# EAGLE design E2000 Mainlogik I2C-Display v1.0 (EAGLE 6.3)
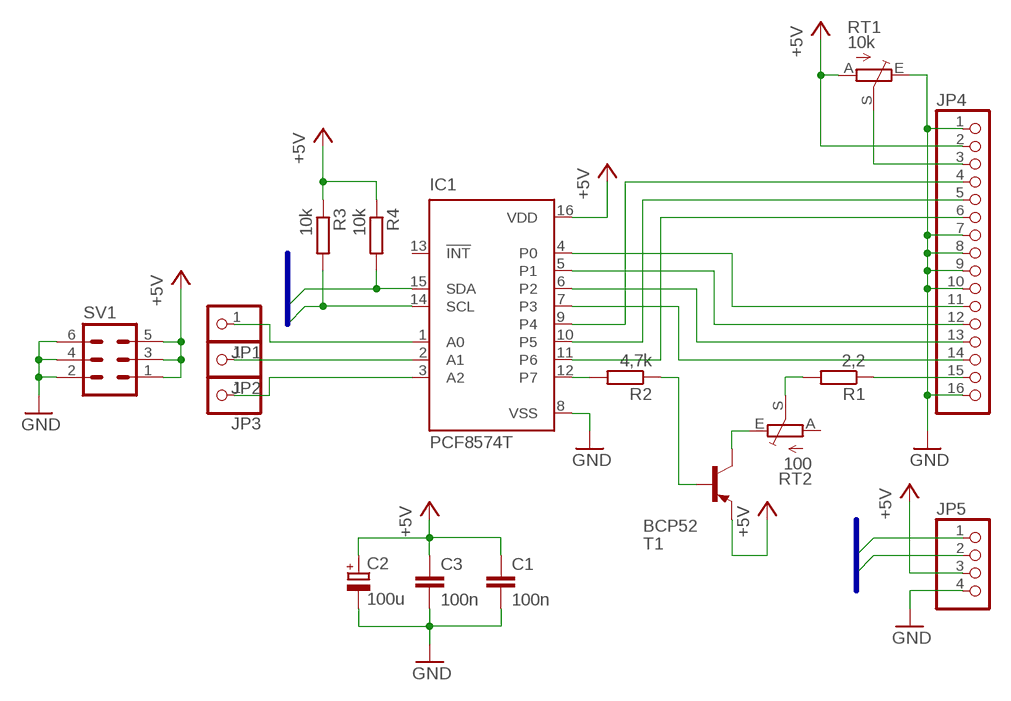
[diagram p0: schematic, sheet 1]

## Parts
C1  100n  C-EUC1206  [C1206]
C2  100u  CPOL-EUD  [PANASONIC_D]
C3  100n  C-EUC1206  [C1206]
IC1  PCF8574T  [SO16W]
JP1  PINHD-1X1  [1X01]
JP2  PINHD-1X1  [1X01]
JP3  PINHD-1X1  [1X01]
JP4  PINHD-1X16  [1X16]
JP5  PINHD-1X4  [1X04]
R1  2,2  R-EU_R1206  [R1206]
R2  4,7k  R-EU_R1206  [R1206]
R3  10k  R-EU_R1206  [R1206]
R4  10k  R-EU_R1206  [R1206]
RT1  10k  TRIM_EU-CA6V  [CA6V]
RT2  100  TRIM_EU-CA6V  [CA6V]
SV1  MA03-2  [MA03-2]
T1  BCP52  [SOT223]

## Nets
+5V: C1.1 C2.+ C3.1 IC1.16(VDD) JP4.2 JP5.3 R3.1 R4.1 RT1.A SV1.1 SV1.3 SV1.5 T1.3(E)
GND: C1.2 C2.- C3.2 IC1.8(VSS) JP4.1 JP4.7 JP4.8 JP4.9 JP4.10 JP4.16 JP5.4 RT1.E SV1.2 SV1.4 SV1.6
N$1: IC1.12(P7) R2.2
N$2: R2.1 T1.1(B)
N$3: RT2.E T1.2(C) T1.4(C)
N$4: R1.2 RT2.S
N$5: JP4.15 R1.1
N$6: IC1.9(P4) JP4.4
N$7: IC1.10(P5) JP4.5
N$8: IC1.11(P6) JP4.6
N$9: IC1.7(P3) JP4.14
N$10: IC1.6(P2) JP4.13
N$11: IC1.5(P1) JP4.12
N$12: IC1.4(P0) JP4.11
N$13: IC1.2(A1) JP2.1
N$14: JP4.3 RT1.S
N$15: IC1.3(A2) JP3.1
N$16: IC1.1(A0) JP1.1
SCL: IC1.14(SCL) JP5.1 R3.2
SDA: IC1.15(SDA) JP5.2 R4.2
Unconnected: IC1.13(!INT) RT2.A

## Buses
SDA,SCL

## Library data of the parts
C1 C3 = rcl:C-EU: CAPACITOR, European symbol
C2 = rcl:CPOL-EU: POLARIZED CAPACITOR, European symbol
IC1 = micro-philips:PCF8574: I2C-Bus Remote 8-bit I/O expander http://www.semiconductors.philips.com/acrobat_download/datasheets/PCF8574_4.pdf; MPN: PCF8574T/3,512; OC_FARNELL: 1201255; OC_NEWARK: 70R6870
JP1-JP3 = pinhead:PINHD-1X1: PIN HEADER
JP4 = pinhead:PINHD-1X16: PIN HEADER
JP5 = pinhead:PINHD-1X4: PIN HEADER
R1-R4 = rcl:R-EU_: RESISTOR, European symbol
RT1 RT2 = pot:TRIM_EU-: POTENTIOMETER
SV1 = con-lstb:MA03-2: PIN HEADER; OC_FARNELL: unknown; OC_NEWARK: unknown
T1 = transistor-pnp:BCP52

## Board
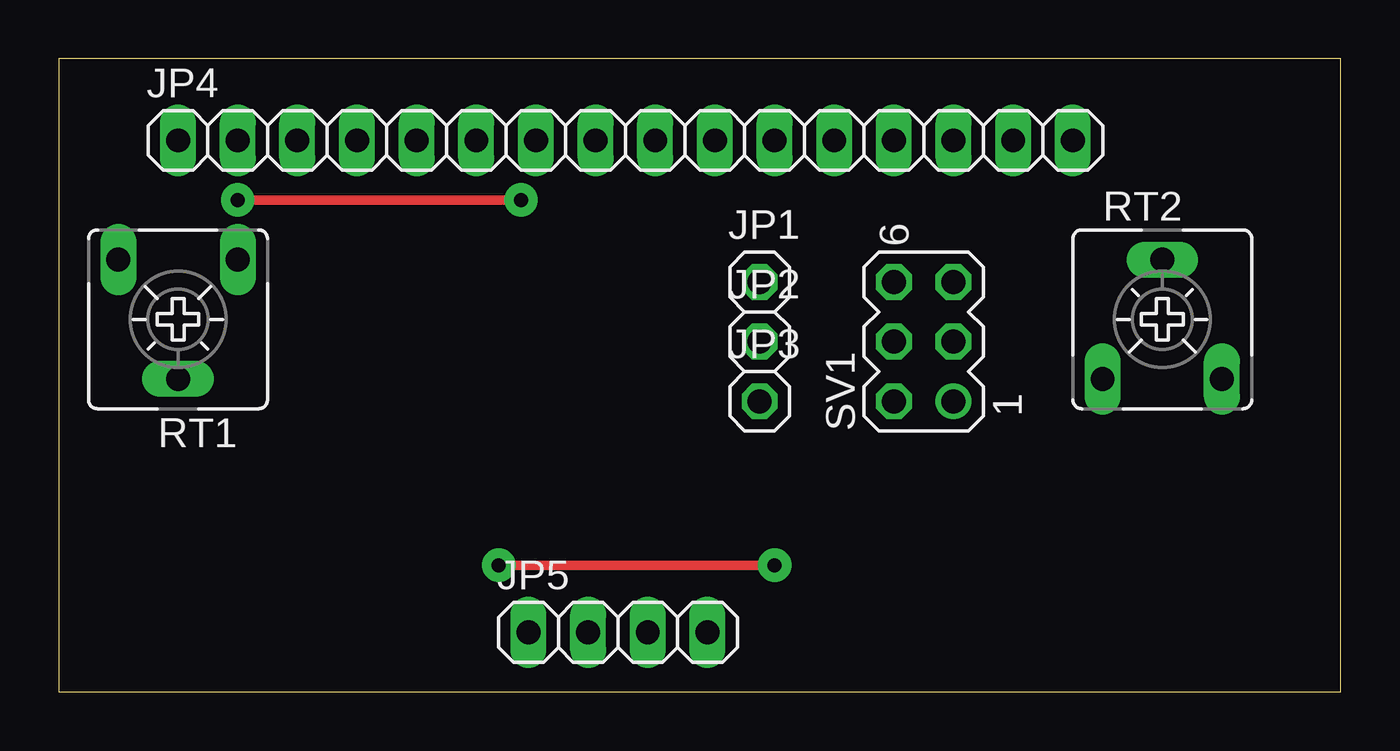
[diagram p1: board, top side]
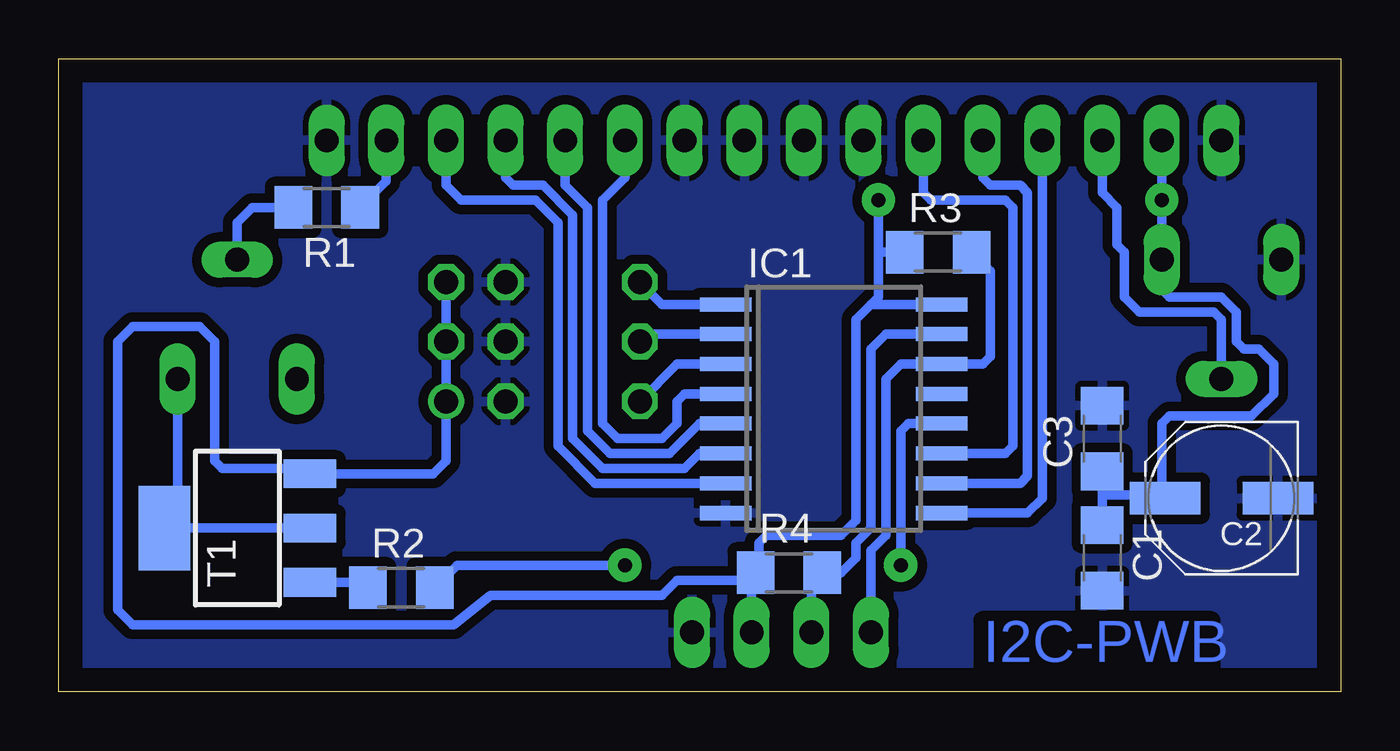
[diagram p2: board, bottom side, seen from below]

Size 54.59 x 26.98 mm. Coordinates in mm from the lower left corner, seen from the top.
Outline: 0,0 54.59,0 54.59,26.98 0,26.98 0,0
Copper layers (1*16): Top 0.035mm / dielectric 1.5mm / Bottom 0.035mm
Design rules "default": minimum track width 10mil, minimum drill 24mil, track to track 8mil, track to pad 8mil, pad to pad 8mil, via to via 8mil, smd to smd 8mil, copper to edge 40mil, drill to drill 8mil, minimum pad ring 10mil, minimum via ring 8mil, stop-mask expansion 4mil, vias tented up to drill 0mil, thermal gap 10mil

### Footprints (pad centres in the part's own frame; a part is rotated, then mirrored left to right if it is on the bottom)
C1206 = smd 1.6 x 1.8: 1 -1.4,0; 2 1.4,0
PANASONIC_D = smd 3 x 1.4: + 2.4,0; - -2.4,0
SO16W = smd 0.6 x 2.2: 1 -4.445,-4.6; 2 -3.175,-4.6; 3 -1.905,-4.6; 4 -0.635,-4.6; 5 0.635,-4.6; 6 1.905,-4.6; 7 3.175,-4.6; 8 4.445,-4.6; 9 4.445,4.6; 10 3.175,4.6; 11 1.905,4.6; 12 0.635,4.6; 13 -0.635,4.6; 14 -1.905,4.6; 15 -3.175,4.6; 16 -4.445,4.6
1X01 = drill 1.016 octagon: 1 0,0
1X16 = drill 1.016 long: 1 -19.05,0; 2 -16.51,0; 3 -13.97,0; 4 -11.43,0; 5 -8.89,0; 6 -6.35,0; 7 -3.81,0; 8 -1.27,0; 9 1.27,0; 10 3.81,0; 11 6.35,0; 12 8.89,0; 13 11.43,0; 14 13.97,0; 15 16.51,0; 16 19.05,0
1X04 = drill 1.016 long: 1 -3.81,0; 2 -1.27,0; 3 1.27,0; 4 3.81,0
R1206 = smd 1.6 x 1.803: 1 -1.422,0; 2 1.422,0
CA6V = drill 1.016 long: A -2.54,-2.54; E 2.54,-2.54; S 0,2.54
MA03-2 = drill 1.016: 1 -2.54,-1.27 | drill 1.016 octagon: 2 -2.54,1.27; 3 0,-1.27; 4 0,1.27; 5 2.54,-1.27; 6 2.54,1.27
SOT223 = smd 1.219 x 2.235: 1 -2.311,-3.099; 2 0,-3.099; 3 2.311,-3.099 | smd 3.6 x 2.2: 4 0,3.099

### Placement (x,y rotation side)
C1  10.16,5.71 270 bottom
C2  5.08,8.26 180 bottom
C3  10.16,10.79 90 bottom
IC1  21.59,12.06 270 bottom
JP1  29.84,17.46 0 top
JP2  29.84,14.92 0 top
JP3  29.84,12.38 0 top
JP4  24.13,23.5 0 top
JP5  23.81,2.54 0 top
R1  43.18,20.64 180 bottom
R2  40.01,4.45 0 bottom
R3  17.14,18.73 0 bottom
R4  23.5,5.08 0 bottom
RT1  5.08,15.88 180 top
RT2  46.99,15.88 0 top
SV1  36.83,14.92 90 top
T1  46.99,6.99 90 bottom

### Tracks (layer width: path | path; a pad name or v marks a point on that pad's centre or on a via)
+5V  (via drill 0.6 pad 1.42)
  Top 0.406: v7.62,20.95 v19.68,20.95
  Bottom 0.406: IC1.16 20,16.51 | 20,16.51 20.64,15.88 20.64,7.3 21.27,6.67 24.45,6.67 24.77,6.35 24.77,5.23 R4.1 25.08,4.92 25.08,4.45 | 20,16.51 19.68,16.83 19.68,18.73 | JP4.2 v7.62,20.95 RT1.A 7.62,17.14 7.3,16.83 5.08,16.83 4.45,16.19 4.45,14.92 4.13,14.61 3.49,14.61 2.86,13.97 2.86,12.7 3.81,11.75 7.3,11.75 7.62,11.43 7.62,8.39 | 7.62,8.39 C2.+ | JP5.3 25.08,4.45 | 25.08,4.45 25.4,4.76 28.26,4.76 28.89,4.13 36.2,4.13 37.78,2.86 51.44,2.86 52.07,3.49 52.07,14.92 51.44,15.56 48.58,15.56 47.94,14.92 47.94,9.84 47.62,9.53 44.12,9.53 T1.3 38.65,9.3 38.1,9.84 SV1.1 SV1.3 SV1.5 | 19.68,18.73 v19.68,20.95 | R3.1 19.68,18.73 | 7.62,8.39 9.98,8.39 10.16,8.57 C3.1 C1.1
GND
  pour Bottom (isolate 0.406): -1.27,27.94 55.88,27.94 55.88,-1.27 -1.27,-1.27
N$1  (via drill 0.6 pad 1.42)
  Top 0.406: v18.73,5.4 v30.48,5.4
  Bottom 0.406: IC1.12 18.41,11.43 18.73,11.11 v18.73,5.4 | v30.48,5.4 37.63,5.4 R2.2
N$2
  Bottom 0.406: T1.1 41.66,4.67 R2.1
N$3
  Bottom 0.406: T1.2 T1.4 49.53,7.7 RT2.E
N$4
  Bottom 0.406: RT2.S 46.99,20 46.35,20.64 R1.2
N$5
  Bottom 0.406: JP4.15 40.64,21.76 R1.1
N$6
  Bottom 0.406: JP4.4 12.7,8.26 13.34,7.62 IC1.9
N$7
  Bottom 0.406: IC1.10 13.65,8.89 13.34,9.21 13.34,21.27 13.65,21.59 14.92,21.59 15.24,21.91 JP4.5
N$8
  Bottom 0.406: IC1.11 14.29,10.16 13.97,10.48 13.97,20.64 14.29,20.95 17.46,20.95 17.78,21.27 JP4.6
N$9
  Bottom 0.406: IC1.7 31.75,8.89 33.34,10.48 33.34,20 34.29,20.95 37.47,20.95 38.1,21.59 JP4.14
N$10
  Bottom 0.406: IC1.6 27.3,10.16 27.94,9.53 31.43,9.53 32.7,10.79 32.7,20.32 33.97,21.59 35.24,21.59 35.56,21.91 JP4.13
N$11
  Bottom 0.406: IC1.5 27.3,11.43 28.57,10.16 31.11,10.16 32.07,11.11 32.07,20.64 33.02,21.59 JP4.12
N$12
  Bottom 0.406: IC1.4 27.94,12.7 28.26,12.38 28.26,11.43 28.89,10.79 30.8,10.79 31.43,11.43 31.43,20.95 30.48,21.91 JP4.11
N$13
  Bottom 0.406: IC1.2 29.53,15.24 JP2.1
N$14
  Bottom 0.406: JP4.3 10.16,21.27 9.53,20.64 9.53,19.05 9.21,18.73 9.21,16.83 8.57,16.19 5.4,16.19 5.08,15.88 RT1.S
N$15
  Bottom 0.406: IC1.3 28.26,13.97 JP3.1
N$16
  Bottom 0.406: IC1.1 28.89,16.51 JP1.1
SCL
  Bottom 0.406: JP5.1 20,6.03 19.37,6.67 19.37,13.34 18.73,13.97 IC1.14 15.24,13.97 14.92,14.29 14.92,17.93 R3.2
SDA
  Bottom 0.406: IC1.15 19.37,15.24 20,14.61 20,6.99 20.64,6.35 20.64,5.71 21.27,5.08 R4.2 22.54,4.61 JP5.2

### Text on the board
Bottom: I2C-PWB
